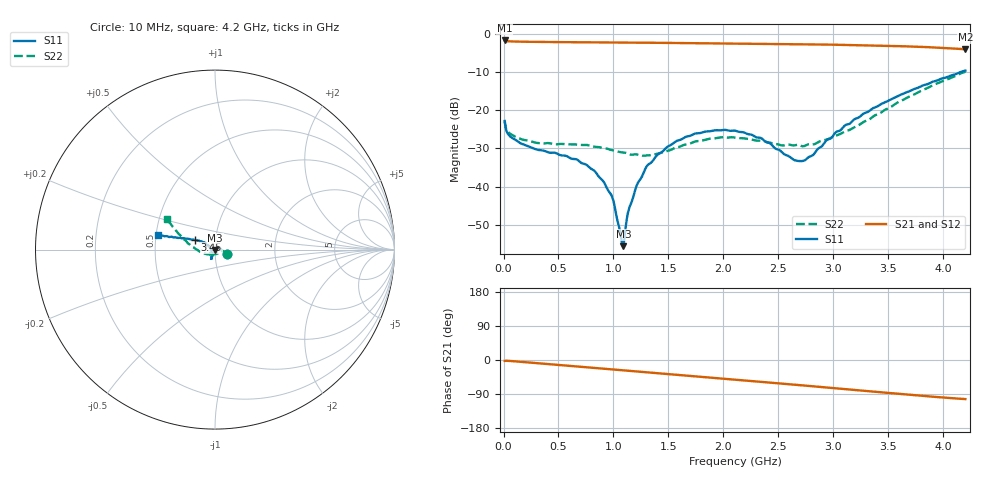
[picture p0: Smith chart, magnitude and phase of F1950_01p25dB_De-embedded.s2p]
! Integrated Device Technology
! Corporate Headquarters
! 6024 Silver Creek Valley Road
! San Jose, CA 95138  USA
! Phone:  1-408-284-8200
! Toll Free:  1-800-223-1366
! Webpage:  http://www.idt.com/
! Timing and RF Division
! 515 Groton Road, Suite 102
! Westford, MA 01886-6024
! Device:  F1950
! Description: 7-bit 0.25 dB Digital Step Attenuator
! Frequency:  150.0 -  4000.00 MHz
! Package:  4x4 mm Thin QFN Plastic Package: 24 pin
! Ports:  2 RF, 12 DC
!  Pin  1  = D0
!  Pin  2  = VDD
!  Pin  3  = Vmode
!  Pin  4  = GND
!  Pin  5  = RF1  =  Port 1
!  Pin  6  = GND
!  Pin  7  = GND
!  Pin  8  = GND
!  Pin  9  = GND
!  Pin 10  = GND
!  Pin 11  = GND
!  Pin 12  = GND
!  Pin 13  = GND
!  Pin 14  = RF2  =  Port 2
!  Pin 15  = GND
!  Pin 16  = LE
!  Pin 17  = CLK
!  Pin 18  = DATE
!  Pin 19  = D6
!  Pin 20  = D5
!  Pin 21  = D4
!  Pin 22  = D3
!  Pin 23  = D2
!  Pin 24  = D1
! State:  5
! Atten State:  1.25 dB
! Voltage:  +5.00 Volts
! Current:  Not Measured mA
! Data:  The device was measured on a the F195X evaluation board which has
!  individual transmission lines to the RF pins.  Data was collected
!  using a calibrated network analyzer.  The evaluation board was
!  de-embedded using a TRL calibration technique.
!  The reference plane is the edge of the package pin.
! Misc:  Board 2019
!  Action Tracker AT0250
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# GHz S dB R 50
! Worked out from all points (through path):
!   420 points, 10 MHz to 4.2 GHz, reference 50 ohm
!   highest |S21| = -1.72 dB at 10 MHz (marker M1); lowest = -4.0 dB at 4.2 GHz (marker M2)
!   group delay of S21, straight-line fit = 68.2 ps
!   lowest |S11| = -55.6 dB at 1.09 GHz (marker M3), VSWR 1.00, Z = 50.1 - j0.137 ohm
!   |S11| at or under -10 dB: start of sweep to 4.155 GHz
!   |S22| runs from -31.9 to -9.9 dB; largest |S21 - S12| = 0.00097
!   S11 on the Smith chart (normalised r, x): 10 MHz: 1.14, -0.06; 3.45 GHz: 0.80, +0.09; 4.2 GHz: 0.51, +0.10
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0.01  -22.82 -21.2  -1.72 -2.3  -1.72 -2.3  -22.70 -20.2
0.06  -26.86 -12.7  -1.96 -2.5  -1.96 -2.5  -26.14 -13.7
0.18  -28.96 -1.9  -2.05 -5.3  -2.04 -5.3  -27.75 -9.3
0.71  -33.86 42.7  -2.19 -18.1  -2.19 -18.1  -29.12 -8.7
0.83  -35.98 45.9  -2.21 -21.0  -2.21 -21.0  -29.57 -15.0
0.97  -41.76 43.6  -2.24 -24.4  -2.24 -24.4  -30.37 -27.1
1  -43.81 42.0  -2.25 -25.1  -2.25 -25.1  -30.52 -30.1
1.07  -53.35 -9.6  -2.26 -26.8  -2.26 -26.8  -31.02 -39.7
1.09  -55.64 -55.9  -2.27 -27.3  -2.27 -27.3  -31.08 -42.3
1.14  -45.99 -94.4  -2.28 -28.5  -2.28 -28.5  -31.49 -49.5
1.21  -39.79 -108.7  -2.29 -30.2  -2.29 -30.2  -31.58 -61.2
1.3  -34.80 -111.8  -2.31 -32.4  -2.31 -32.4  -31.85 -77.5
1.41  -31.45 -112.1  -2.34 -35.0  -2.34 -35.1  -31.34 -96.8
1.74  -26.15 -112.4  -2.42 -43.1  -2.42 -43.1  -28.21 -135.3
2.11  -25.39 -112.5  -2.53 -52.1  -2.53 -52.1  -27.21 -151.0
2.34  -27.28 -117.5  -2.60 -57.7  -2.59 -57.7  -27.98 -151.2
2.66  -33.21 -158.1  -2.69 -65.5  -2.69 -65.5  -29.12 -140.9
2.81  -31.84 165.0  -2.75 -69.3  -2.75 -69.3  -28.96 -138.7
3.11  -23.89 146.9  -2.88 -76.9  -2.87 -76.9  -25.53 -151.3
3.45  -18.17 154.2  -3.09 -85.6  -3.08 -85.7  -20.27 -178.3
3.51  -17.35 155.4  -3.13 -87.1  -3.12 -87.2  -19.36 178.2
4.2  -9.60 165.3  -4.04 -103.1  -4.03 -103.2  -9.91 147.3
